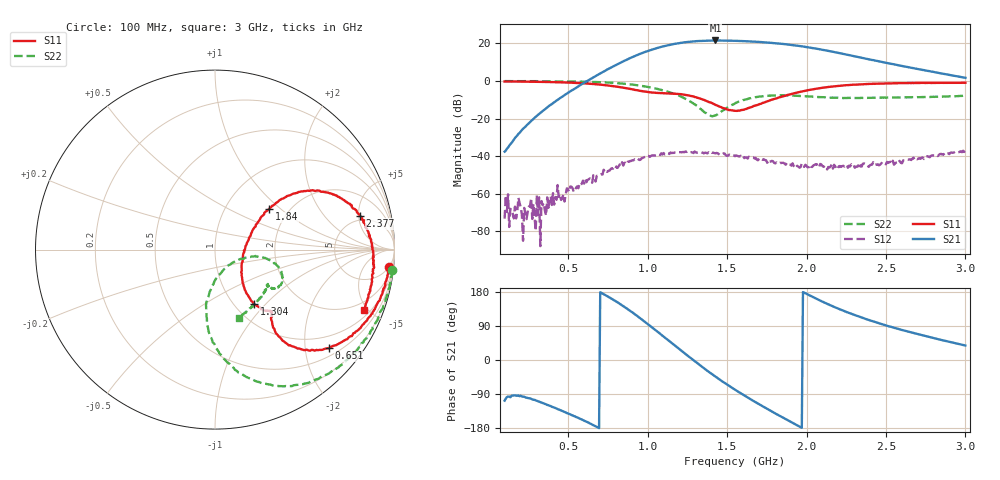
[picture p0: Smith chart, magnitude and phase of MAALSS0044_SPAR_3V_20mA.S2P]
!Part No: MAALSS0044
!Bias: Vdd=3V, Idd=20mA (R1=39ohm)
!2-port de-embedded S-parameters
!Date: Wed Sep 14 15:55:24 2011
!Temp: +25c
!REF Task A17L_2309
!Fixture: 25050XX Rev00
!Test System: Agilent Technologies,E5071C,MY46106711,A.09.61
!Data & Calibration Information:
!Freq	S11:SOLT2(ON)	S21:SOLT2(ON)	S12:SOLT2(ON)	S22:SOLT2(ON)
!PortZ  Port1:50+j0  Port2:50+j0
# Hz S dB R 50
!Freq(Hz)	S11(dB) 	S11(Angle)	S21(dB) 	S21(Angle)	S12(dB) 	S12(Angle)	S22(dB) 	S22(Angle)
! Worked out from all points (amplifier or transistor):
!   401 points, 100 MHz to 3 GHz, reference 50 ohm
!   highest |S21| = 21.6 dB at 1.427 GHz (marker M1)
!   |S21| within 3 dB of that: 1.106 GHz to 1.961 GHz (855.6 MHz wide, 55.8 % of centre)
!   unconditionally stable (mu >= 1): start of sweep to end of sweep
!   at 578.5 MHz: K = 7.36, MAG = 15.1 dB, |S12| = -55.5 dB
!   at 1.55 GHz: K = 3.95, MAG = 21.9 dB, |S12| = -40.1 dB
!   at 3 GHz: K = 4.49, MAG = 9.8 dB, |S12| = -36.9 dB
!   S11 on the Smith chart (normalised r, x): 100 MHz: 5, -18; 651 MHz: 0.68, -2.52; 1.304 GHz: 1.23, -0.85; 1.84 GHz: 1.59, +0.84; 2.377 GHz: 4.34, +5.18; 3 GHz: 1.40, -4.76
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1e8  -0.24 -5.9  -37.68 -107.3  -73.40 92.0  -0.05 -6.5
5.8575e8  -1.19 -36.4  -1.71 -157.0  -54.73 179.3  -0.36 -39.6
6.51e8  -1.53 -40.9  1.55 -170.5  -54.24 167.9  -0.48 -45.0
7.8875e8  -2.81 -49.6  8.00 157.8  -46.03 152.9  -1.01 -57.5
9.0475e8  -4.45 -53.8  12.76 125.7  -42.24 134.2  -1.95 -69.3
9.845e8  -5.65 -52.3  15.51 100.1  -40.48 117.3  -2.91 -77.3
1.0715e9  -6.43 -48.7  17.86 71.8  -39.13 98.6  -4.48 -85.9
1.18025e9  -6.85 -48.7  19.96 35.4  -37.99 77.3  -7.23 -95.2
1.2455e9  -7.53 -52.2  20.76 13.4  -37.83 63.9  -9.82 -98.9
1.3035e9  -8.62 -54.2  21.25 -5.5  -38.05 49.1  -12.84 -96.3
1.35425e9  -10.07 -54.2  21.48 -21.7  -38.64 35.8  -16.47 -84.8
1.42675e9  -12.70 -48.6  21.62 -43.7  -38.58 24.8  -18.40 -38.6
1.492e9  -14.92 -34.3  21.59 -62.3  -39.62 7.4  -14.74 -13.9
1.55e9  -15.91 -13.4  21.44 -78.3  -40.09 -5.8  -11.94 -9.4
1.68775e9  -12.85 25.3  20.88 -113.3  -42.03 -30.2  -8.49 -16.2
1.84e9  -8.50 36.9  19.85 -149.5  -43.78 -67.2  -7.63 -27.4
1.93425e9  -6.31 36.8  18.91 -171.1  -44.66 -90.3  -7.88 -31.2
2.03575e9  -4.54 33.4  17.65 167.2  -45.84 -116.4  -8.32 -34.5
2.18075e9  -2.78 24.9  15.29 138.8  -45.51 -151.0  -8.91 -34.3
2.3765e9  -1.63 13.1  11.89 107.8  -44.62 -156.9  -8.98 -34.9
2.5215e9  -1.25 5.0  9.35 88.5  -43.23 -164.0  -8.83 -39.7
3e9  -0.95 -21.9  1.70 38.2  -36.94 -170.9  -7.85 -71.0
